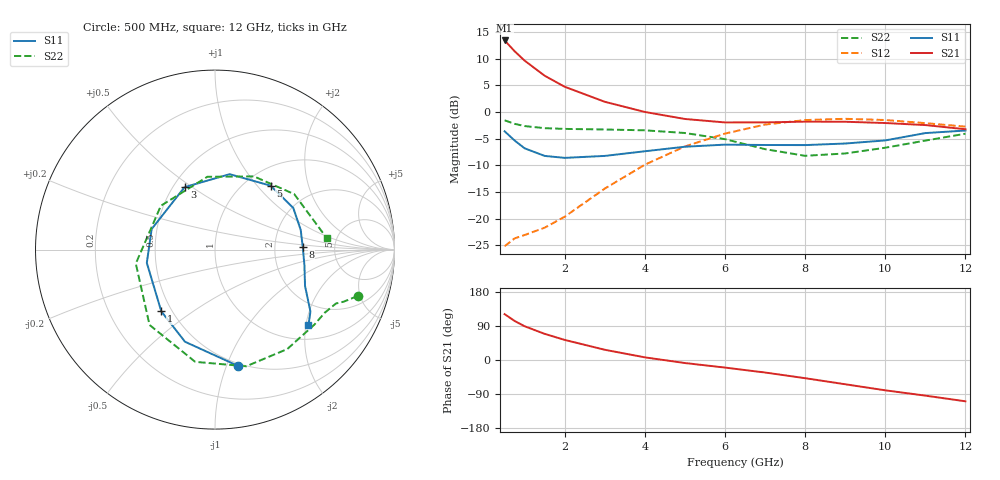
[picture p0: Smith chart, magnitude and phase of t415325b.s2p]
!AT-41532
!S-PARAMETERS at Vce=5V  Ic=2mA.  LAST UPDATED 05-29-98
# ghz s ma r 50
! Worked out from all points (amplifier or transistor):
!   15 points, 500 MHz to 12 GHz, reference 50 ohm
!   highest |S21| = 13.4 dB at 500 MHz (marker M1)
!   |S21| within 3 dB of that: start of sweep to 887.9 MHz
!   unconditionally stable (mu >= 1): 1.383 GHz to 2.282 GHz; 11.54 GHz to end of sweep
!   at 1 GHz: K = 0.83, MSG = 16.4 dB, |S12| = -23.1 dB
!   at 5 GHz: K = 0.73, MSG = 2.6 dB, |S12| = -6.5 dB
!   at 12 GHz: K = 1.00, MAG = -0.6 dB, |S12| = -2.7 dB
!   lowest NFmin = 1.20 dB at 900 MHz
!   S11 on the Smith chart (normalised r, x): 500 MHz: 0.48, -1.09; 1 GHz: 0.44, -0.38; 3 GHz: 0.57, +0.47; 5 GHz: 1.29, +1.18; 8 GHz: 2.91, +0.13; 12 GHz: 1.35, -2.07
0.5  0.659 -79.0  4.696 121.0  0.055 53.0  0.836 -18.0
0.75  0.54 -108.0  3.72 103.0  0.065 48.0  0.774 -22.0
1  0.456 -131.0  3.034 89.0  0.07 48.0  0.738 -24.0
1.5  0.387 -169.0  2.19 69.0  0.082 55.0  0.705 -30.0
2  0.371 162.0  1.726 53.0  0.104 63.0  0.694 -37.0
3  0.387 116.0  1.247 27.0  0.191 67.0  0.685 -54.0
4  0.428 79.0  1.001 7.0  0.32 56.0  0.673 -75.0
5  0.472 49.0  0.86 -8.0  0.475 38.0  0.635 -100.0
6  0.494 28.0  0.798 -20.0  0.627 17.0  0.556 -131.0
7  0.49 13.0  0.799 -33.0  0.762 -5.0  0.448 -170.0
8  0.489 2.0  0.812 -48.0  0.84 -29.0  0.388 141.0
9  0.506 -10.0  0.81 -64.0  0.863 -51.0  0.408 96.0
10  0.541 -22.0  0.788 -80.0  0.841 -71.0  0.462 62.0
11  0.634 -33.0  0.754 -94.0  0.786 -90.0  0.539 35.0
12  0.67 -39.0  0.689 -109.0  0.729 -105.0  0.625 6.0
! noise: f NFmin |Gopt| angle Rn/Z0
0.9  1.2  0.35  100  0.17
1.8  1.5  0.48  178  0.07
2  1.6  0.51  -166  0.07
2.5  1.9  0.6  -137  0.18
3  2.2  0.65  -112  0.43
3.5  2.5  0.7  -92  0.89
4  2.9  0.74  -73  1.59
